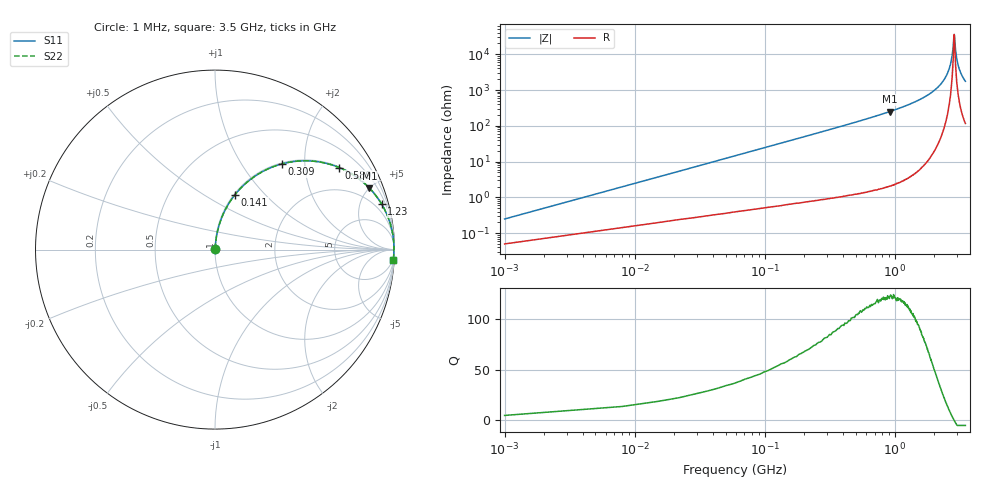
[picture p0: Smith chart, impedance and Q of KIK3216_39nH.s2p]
!version-2
!date-01.2022
!Series
# MHz S RI R 50
!Freq ReS11 ImS11 ReS21 ImS21 ReS12 ImS12 ReS22 ImS22
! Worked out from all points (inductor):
!   501 points, 1 MHz to 3.5 GHz, reference 50 ohm
!   read as one part in series: L = 39 nH near 15 MHz
!   highest Q = 122 at 918 MHz (marker M1), where L = 43.4 nH
!   self-resonance near 2.865 GHz
!   S11 on the Smith chart (normalised r, x): 1 MHz: 1.00, +0.00; 141 MHz: 1.01, +0.69; 309 MHz: 1.02, +1.53; 589 MHz: 1.03, +3.01; 1.23 GHz: 1.07, +7.35; 3.5 GHz: 3, -35
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1  0.000517 0.00245  0.9995 -0.00245  0.9995 -0.00245  0.000517 0.00245
22  0.00527 0.0535  0.9947 -0.0535  0.9947 -0.0535  0.00527 0.0535
36  0.0107 0.087  0.9893 -0.087  0.9893 -0.087  0.0107 0.087
78  0.0393 0.1829  0.9607 -0.1829  0.9607 -0.1829  0.0393 0.1829
141  0.1114 0.3059  0.8886 -0.3059  0.8886 -0.3059  0.1114 0.3059
309  0.3714 0.4772  0.6286 -0.4772  0.6286 -0.4772  0.3714 0.4772
589  0.6926 0.4569  0.3074 -0.4569  0.3074 -0.4569  0.6926 0.4569
918  0.8606 0.3423  0.1394 -0.3423  0.1394 -0.3423  0.8606 0.3423
1170  0.9201 0.2669  0.0799 -0.2669  0.0799 -0.2669  0.9201 0.2669
1230  0.9291 0.2522  0.0708 -0.2522  0.0708 -0.2522  0.9291 0.2522
1760  0.9775 0.1415  0.0225 -0.1415  0.0225 -0.1415  0.9775 0.1415
2340  0.9944 0.0581  0.00564 -0.0581  0.00564 -0.0581  0.9944 0.0581
2540  0.9963 0.0352  0.00366 -0.0352  0.00366 -0.0352  0.9963 0.0352
2680  0.997 0.0199  0.00296 -0.0199  0.00296 -0.0199  0.997 0.0199
2770  0.9972 0.0104  0.00278 -0.0104  0.00278 -0.0104  0.9972 0.0104
2865  0.9972 0.000588  0.00279 -0.000588  0.00279 -0.000588  0.9972 0.000588
2880  0.9972 -0.000791  0.00281 0.000791  0.00281 0.000791  0.9972 -0.000791
2920  0.9971 -0.00489  0.00289 0.00489  0.00289 0.00489  0.9971 -0.00489
3000  0.9969 -0.0129  0.00314 0.0129  0.00314 0.0129  0.9969 -0.0129
3100  0.9964 -0.022  0.0036 0.022  0.0036 0.022  0.9964 -0.022
3290  0.9951 -0.0387  0.00491 0.0387  0.00491 0.0387  0.9951 -0.0387
3500  0.9931 -0.0562  0.00693 0.0562  0.00693 0.0562  0.9931 -0.0562
